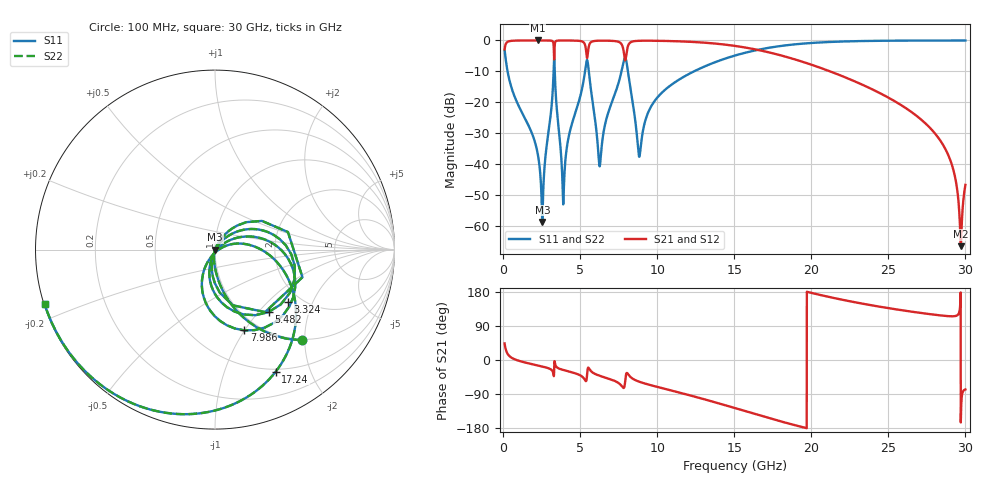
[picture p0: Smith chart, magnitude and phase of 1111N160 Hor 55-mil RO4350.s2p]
# GHz S MA R 50
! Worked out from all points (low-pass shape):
!   3201 points, 100 MHz to 30 GHz, reference 50 ohm
!   highest |S21| = -0.01 dB at 2.258 GHz (marker M1); lowest = -66.7 dB at 29.7 GHz (marker M2)
!   |S21| within 3 dB of the highest: start of sweep to 3.295 GHz; 8.045 GHz to 16.47 GHz (8.428 GHz wide, 68.8 % of centre)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
!   lowest |S11| = -58.8 dB at 2.548 GHz (marker M3), VSWR 1.00, Z = 50.1 - j0.021 ohm
!   |S11| at or under -10 dB: 291.3 MHz to 3.279 GHz (2.987 GHz wide, 167 % of centre); 5.563 GHz to 7.685 GHz (2.122 GHz wide, 32 % of centre); 8.102 GHz to 12.4 GHz (4.295 GHz wide, 41.9 % of centre)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
!   |S22| runs from -58.8 to 0.0 dB; largest |S21 - S12| = 0
!   S11 on the Smith chart (normalised r, x): 100 MHz: 0.98, -1.93; 3.324 GHz: 1.72, -1.32; 5.482 GHz: 1.29, -1.13; 7.986 GHz: 0.85, -1.00; 17.24 GHz: 0.47, -1.51; 30 GHz: 0.00, -0.16
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0.1  0.699 -46.3  0.7149 43.7  0.7149 43.7  0.699 -46.3
0.511125  0.1838 -82.8  0.9825 7.1  0.9825 7.1  0.1838 -82.8
2.258406  0.01414 -100.8  0.9987 -14.5  0.9987 -14.5  0.01414 -100.8
2.548062  0.00115 -10.5  0.9986 -17.3  0.9986 -17.3  0.00115 -10.5
3.323594  0.4979 -35.5  0.5269 -10.1  0.5269 -10.1  0.4979 -35.5
3.921594  0.002625 7.3  0.9974 -26.5  0.9974 -26.5  0.002625 7.3
4.286  0.02967 54.8  0.9966 -30.5  0.9966 -30.5  0.02967 54.8
5.089563  0.1503 40.3  0.9696 -42.6  0.9696 -42.6  0.1503 40.3
5.482  0.4583 -49.4  0.5621 -26.0  0.5621 -26.0  0.4583 -49.4
6.276219  0.009199 -28.9  0.9903 -41.6  0.9903 -41.6  0.009199 -28.9
7.575  0.243 16.4  0.9273 -63.5  0.9273 -63.5  0.243 16.4
7.986125  0.4783 -70.1  0.5639 -36.9  0.5639 -36.9  0.4783 -70.1
8.836406  0.01303 -50.0  0.9861 -57.3  0.9861 -57.3  0.01303 -50.0
10.06978  0.1236 15.8  0.9856 -71.6  0.9856 -71.6  0.1236 15.8
15.05  0.5693 -37.5  0.8146 -126.9  0.8146 -126.9  0.5693 -37.5
17.23644  0.7591 -63.5  0.6419 -153.0  0.6419 -153.0  0.7591 -63.5
20.03956  0.9103 -93.7  0.4019 176.8  0.4019 176.8  0.9103 -93.7
25.01978  0.9893 -133.8  0.1178 136.8  0.1178 136.8  0.9893 -133.8
28.57041  0.9963 -154.8  0.01994 116.8  0.01994 116.8  0.9963 -154.8
29.27119  0.9965 -158.5  0.007115 115.6  0.007115 115.6  0.9965 -158.5
29.701  0.9966 -160.7  0.0004649 -164.7  0.0004649 -164.7  0.9966 -160.7
30  0.9965 -162.2  0.00457 -77.7  0.00457 -77.7  0.9965 -162.2
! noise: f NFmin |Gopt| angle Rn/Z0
0.1  0.0007942  0.7757  2.53  0.0007234
3.417  0.03684  0.8292  23.21  0.0436
6.743  0.03026  0.6418  44.13  0.01382
10.06  0.03239  0.545  63.11  0.009495
13.39  0.03714  0.5093  76.97  0.008596
16.7  0.05306  0.5867  91.22  0.01229
20.03  0.08601  0.7103  107.9  0.02133
23.35  0.1664  0.8383  126.5  0.04547
26.67  0.4647  0.9391  145.1  0.1553
30  5.996  0.9943  162.2  7.862
